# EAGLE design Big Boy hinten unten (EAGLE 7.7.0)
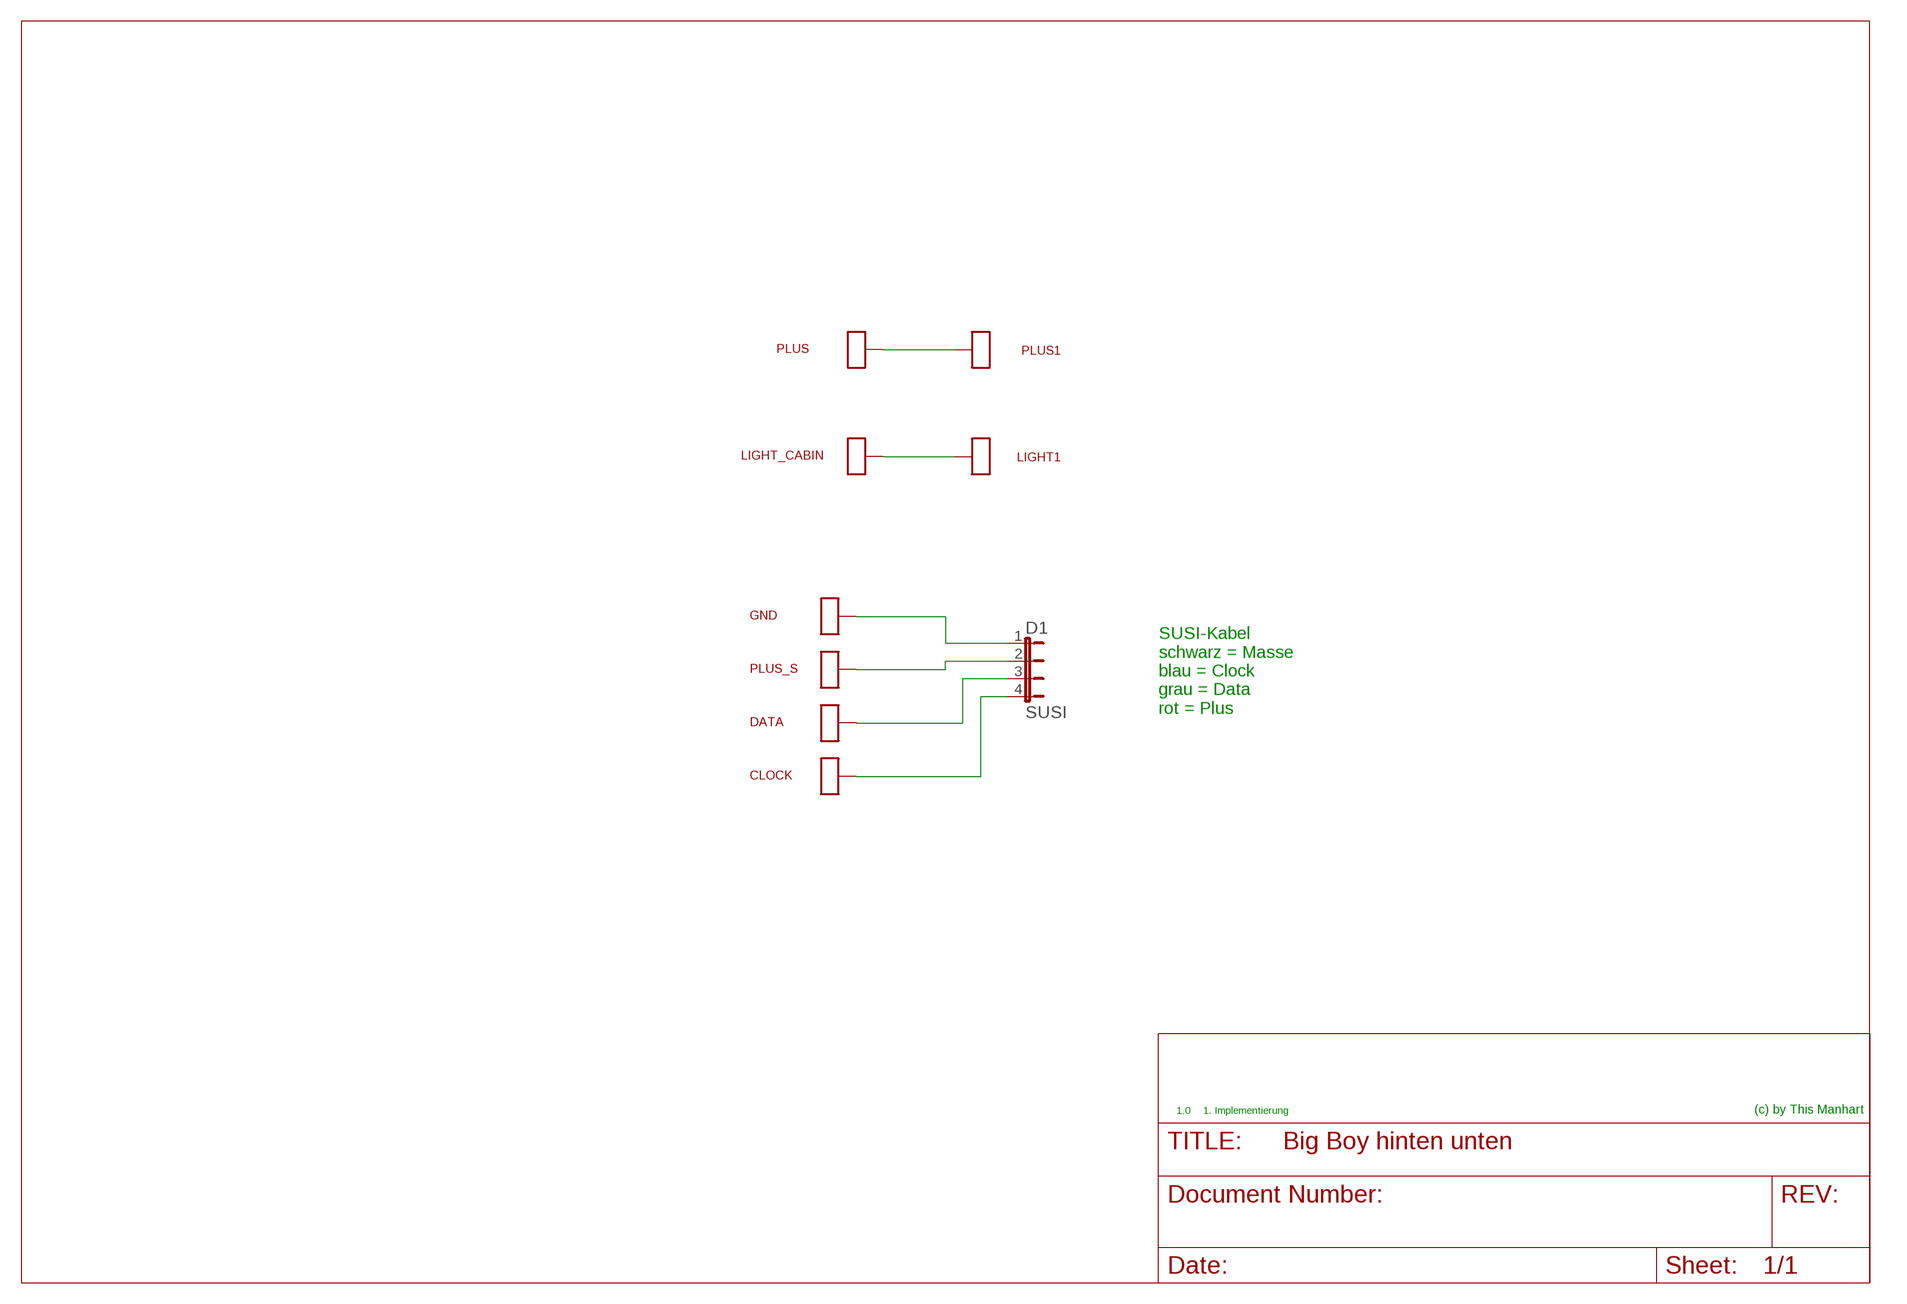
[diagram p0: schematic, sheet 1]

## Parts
CLOCK  SMD_LOETPADKLEIN  [SMD_LOETPAD]
D1  SUSI  JUMPER_4P  [JUMPER_4P_2.54_QUAD_OHNE]
DATA  SMD_LOETPADKLEIN  [SMD_LOETPAD]
GND  SMD_LOETPADKLEIN  [SMD_LOETPAD]
LIGHT1  SMD_LOETPADKLEIN  [SMD_LOETPAD]
LIGHT_CABIN  SMD_LOETPAD  [SMD_LOETPAD_XL]
PLUS  SMD_LOETPAD  [SMD_LOETPAD_XL]
PLUS1  SMD_LOETPADKLEIN  [SMD_LOETPAD]
PLUS_S  SMD_LOETPADKLEIN  [SMD_LOETPAD]

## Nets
N$1: PLUS1.P$1 PLUS.P$1
N$2: LIGHT1.P$1 LIGHT_CABIN.P$1
N$3: D1.1 GND.P$1
N$4: D1.2 PLUS_S.P$1
N$5: D1.3 DATA.P$1
N$6: CLOCK.P$1 D1.4

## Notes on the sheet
- SUSI-Kabel
  schwarz = Masse
  blau = Clock
  grau = Data
  rot = Plus
- 1.0 | 1. Implementierung | (c) by This Manhart

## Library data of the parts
CLOCK DATA GND LIGHT1 LIGHT_CABIN PLUS PLUS1 PLUS_S = 0_mm:SMD_LOETPAD
D1 = 0_mm:JUMPER_4P

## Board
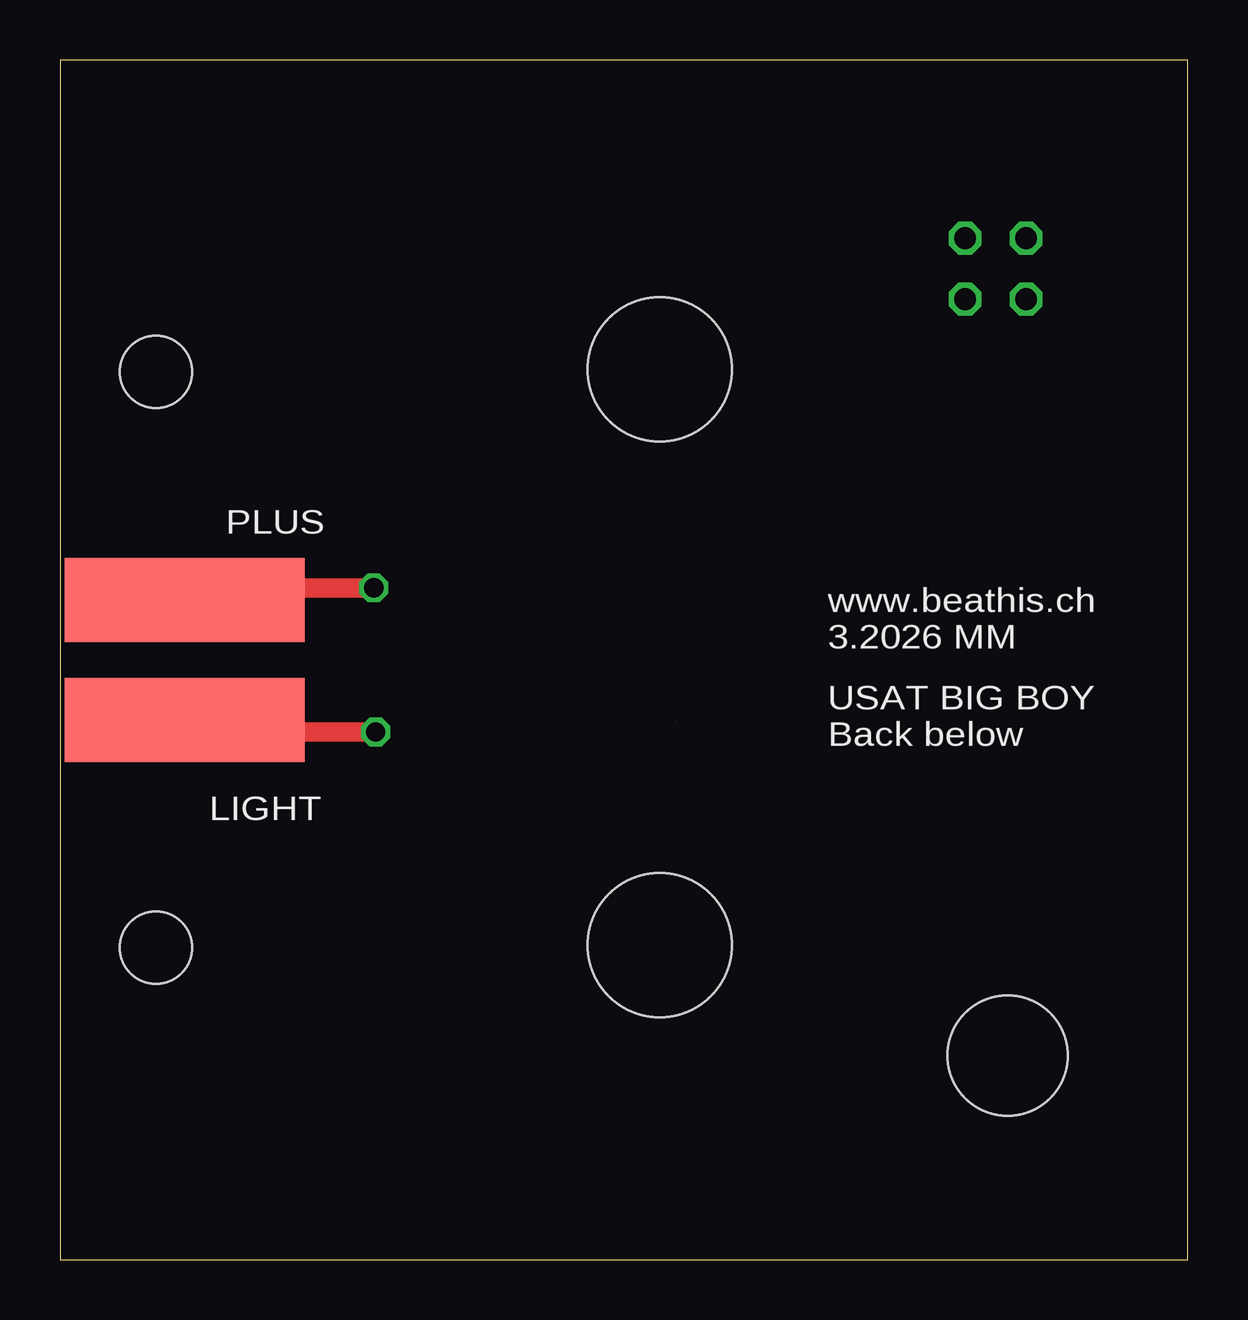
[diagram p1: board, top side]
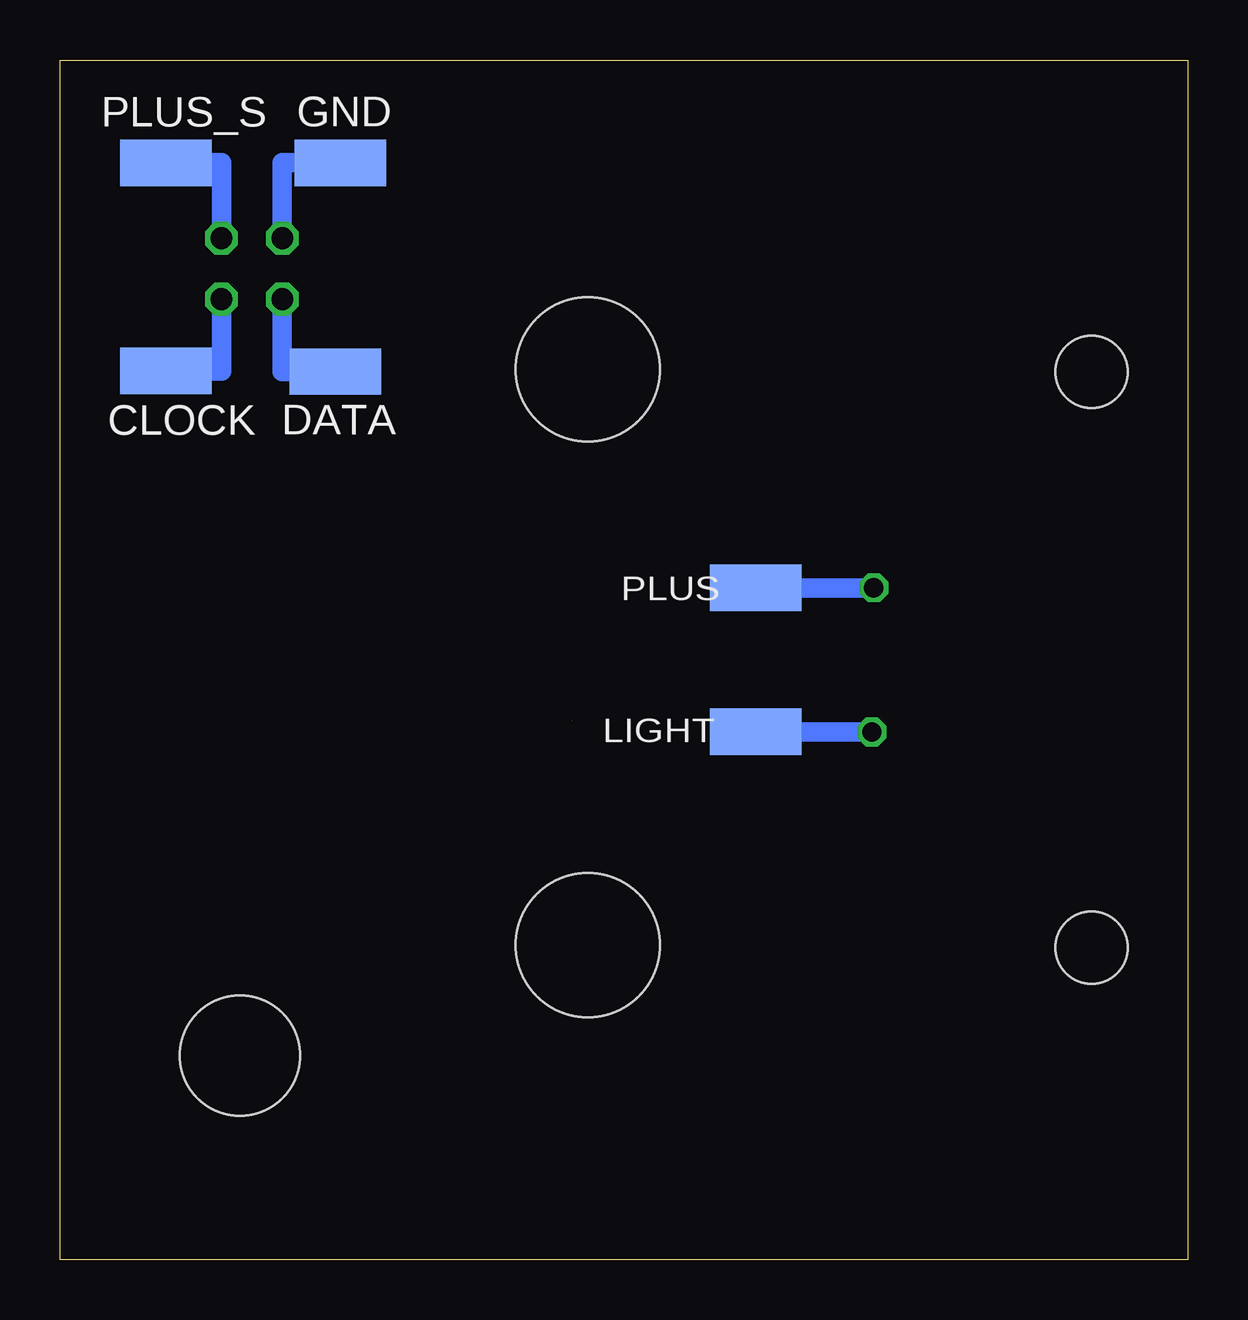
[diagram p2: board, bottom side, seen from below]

Size 47 x 50 mm. Coordinates in mm from the lower left corner, seen from the top.
Outline: 25.65,22.45 25.66,22.45
Outline: 47,0 47,50 0,50 0,0 47,0
Copper layers (1*16): Top 0.035mm / dielectric 1.5mm / Bottom 0.035mm
Design rules "pcb-pool": minimum track width 6mil, minimum drill 12mil, track to track 6mil, track to pad 6mil, pad to pad 6mil, via to via 6mil, smd to smd 8mil, copper to edge 40mil, drill to drill 20mil, minimum pad ring 8mil, minimum via ring 8mil, stop-mask expansion 6mil, vias tented up to drill 0mil, thermal gap 10mil
Holes 3 mm at 4,13 4,37
Holes 6 mm at 25,37.1 25,13.1
Holes 5 mm at 39.5,8.5

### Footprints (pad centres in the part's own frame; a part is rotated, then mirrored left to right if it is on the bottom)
SMD_LOETPAD = smd 3.81 x 1.93: P$1 0,0
JUMPER_4P_2.54_QUAD_OHNE = drill 0.914 octagon: 1 -1.27,-1.27; 2 -1.27,1.27; 3 1.27,-1.27; 4 1.27,1.27
SMD_LOETPAD_XL = smd 10 x 3.5: P$1 0,0

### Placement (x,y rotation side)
CLOCK  42.59,37.04 0 bottom
D1  39,41.3 270 top
DATA  35.52,37.01 0 bottom
GND  35.31,45.71 0 bottom
LIGHT1  18,22 0 bottom
LIGHT_CABIN  5.2,22.5 0 top
PLUS  5.2,27.5 180 top
PLUS1  18,28 0 bottom
PLUS_S  42.59,45.71 0 bottom

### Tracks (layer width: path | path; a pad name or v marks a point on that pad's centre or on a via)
N$1  (via drill 0.8 pad 1.2)
  Top 0.813: v13.08,28 7.5,28 7.5,27.82 PLUS.P$1
  Bottom 0.813: PLUS1.P$1 v13.08,28
N$2  (via drill 0.8 pad 1.2)
  Top 0.813: LIGHT_CABIN.P$1 7.95,22.37 7.95,22 v13.16,22 v13.16,21.99
  Bottom 0.813: v13.16,21.99 LIGHT1.P$1
N$3
  Bottom 0.813: GND.P$1 37.73,45.71 D1.1
N$4
  Bottom 0.813: D1.2 40.27,45.71 PLUS_S.P$1
N$5
  Bottom 0.813: DATA.P$1 37.73,37.01 D1.3
N$6
  Bottom 0.813: D1.4 40.27,37.04 CLOCK.P$1

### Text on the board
tNames: PLUS | www.beathis.ch / 3.2026 MM | USAT BIG BOY / Back below | LIGHT
bNames: PLUS | LIGHT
